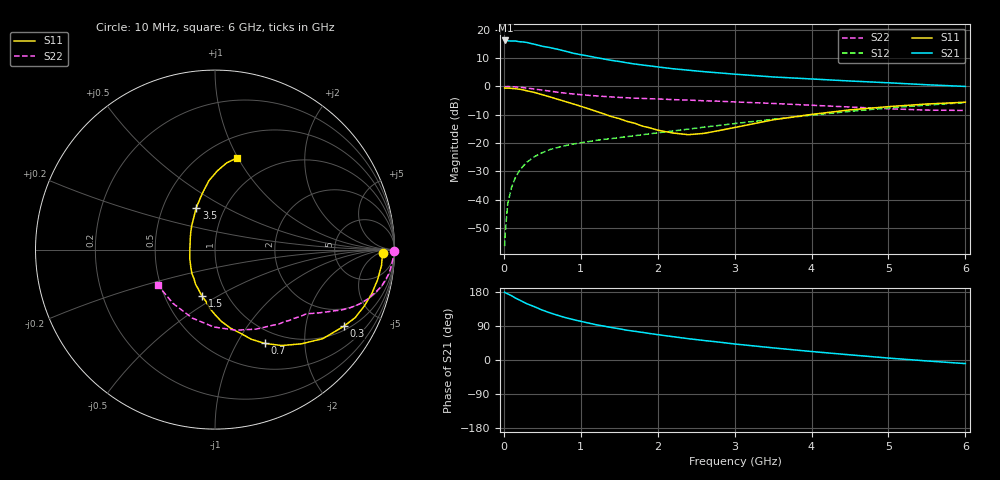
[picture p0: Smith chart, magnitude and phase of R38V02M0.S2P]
! SIEMENS Small Signal Semiconductors
! BFR181
! Si NPN RF Bipolar Junction Transistor in SOT23
! VCE = 8 V  IC = 2 mA
! Common Emitter S-Parameters:  May  1996
# GHz  S  MA  R  50
!  f  S11  S21  S12  S22
! GHz  MAG  ANG  MAG  ANG  MAG  ANG  MAG  ANG
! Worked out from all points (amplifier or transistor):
!   36 points, 10 MHz to 6 GHz, reference 50 ohm
!   highest |S21| = 16.2 dB at 20 MHz (marker M1)
!   |S21| within 3 dB of that: start of sweep to 680.8 MHz
!   unconditionally stable (mu >= 1): 1.648 GHz to 3.477 GHz
!   at 250 MHz: K = 0.22, MSG = 22.0 dB, |S12| = -28.2 dB
!   at 1.4 GHz: K = 0.93, MSG = 13.8 dB, |S12| = -18.5 dB
!   at 6 GHz: K = 0.86, MSG = 2.9 dB, |S12| = -5.8 dB
!   lowest NFmin = 1.35 dB at 450 MHz
!   S11 on the Smith chart (normalised r, x): 10 MHz: 27, -9; 300 MHz: 1.15, -3.25; 700 MHz: 0.82, -1.31; 1.5 GHz: 0.76, -0.43; 3.5 GHz: 0.73, +0.37; 6 GHz: 0.70, +0.99
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0.01  0.9353 -1.2  6.386 178.8  0.0015 91.4  0.9968 -0.5
0.02  0.933 -2.1  6.471 177.4  0.0028 90.3  0.9865 -1.1
0.05  0.9318 -5.5  6.378 174.6  0.0083 86.5  0.9942 -2.6
0.1  0.921 -10.6  6.325 169.7  0.0164 84.3  0.9872 -5.0
0.15  0.9072 -15.7  6.322 163.5  0.0245 80.7  0.9785 -7.8
0.3  0.8347 -30.8  5.954 148.4  0.0457 72.2  0.9325 -14.2
0.4  0.7796 -39.5  5.533 140.5  0.0575 67.5  0.8959 -17.8
0.5  0.7122 -47.5  5.116 131.7  0.0674 63.6  0.8594 -20.7
0.6  0.6509 -55.2  4.838 124.4  0.0764 60.7  0.8227 -23.1
0.7  0.5912 -62.1  4.522 117.9  0.0831 58.5  0.7884 -25.1
0.8  0.5386 -68.0  4.183 111.9  0.0897 56.8  0.7586 -26.6
0.9  0.4897 -72.8  3.858 106.7  0.0956 55.3  0.7333 -27.9
1.1  0.4019 -84.9  3.428 97.6  0.1056 54.1  0.6946 -30.2
1.3  0.3264 -95.4  3.043 89.4  0.1157 53.6  0.6635 -32.1
1.5  0.2691 -105.7  2.752 82.4  0.1242 53.9  0.6383 -33.9
1.9  0.1847 -134.2  2.299 69.8  0.1452 54.6  0.6047 -37.8
2.2  0.1496 -160.0  2.047 61.5  0.1629 55.4  0.5832 -41.1
2.6  0.1475 159.6  1.817 51.5  0.1902 55.6  0.5564 -46.3
3.5  0.2559 114.1  1.466 32.0  0.2623 52.8  0.499 -62.6
4.5  0.3845 95.2  1.243 13.6  0.3612 45.2  0.4312 -90.9
5.5  0.488 82.3  1.067 -2.5  0.4669 33.1  0.3804 -127.9
6  0.5244 76.5  0.997 -9.5  0.5158 26.1  0.375 -148.3
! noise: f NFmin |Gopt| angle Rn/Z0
0.45  1.35  0.6  17  0.4
0.9  1.45  0.5  36  0.4
1.8  1.8  0.31  80  0.37
